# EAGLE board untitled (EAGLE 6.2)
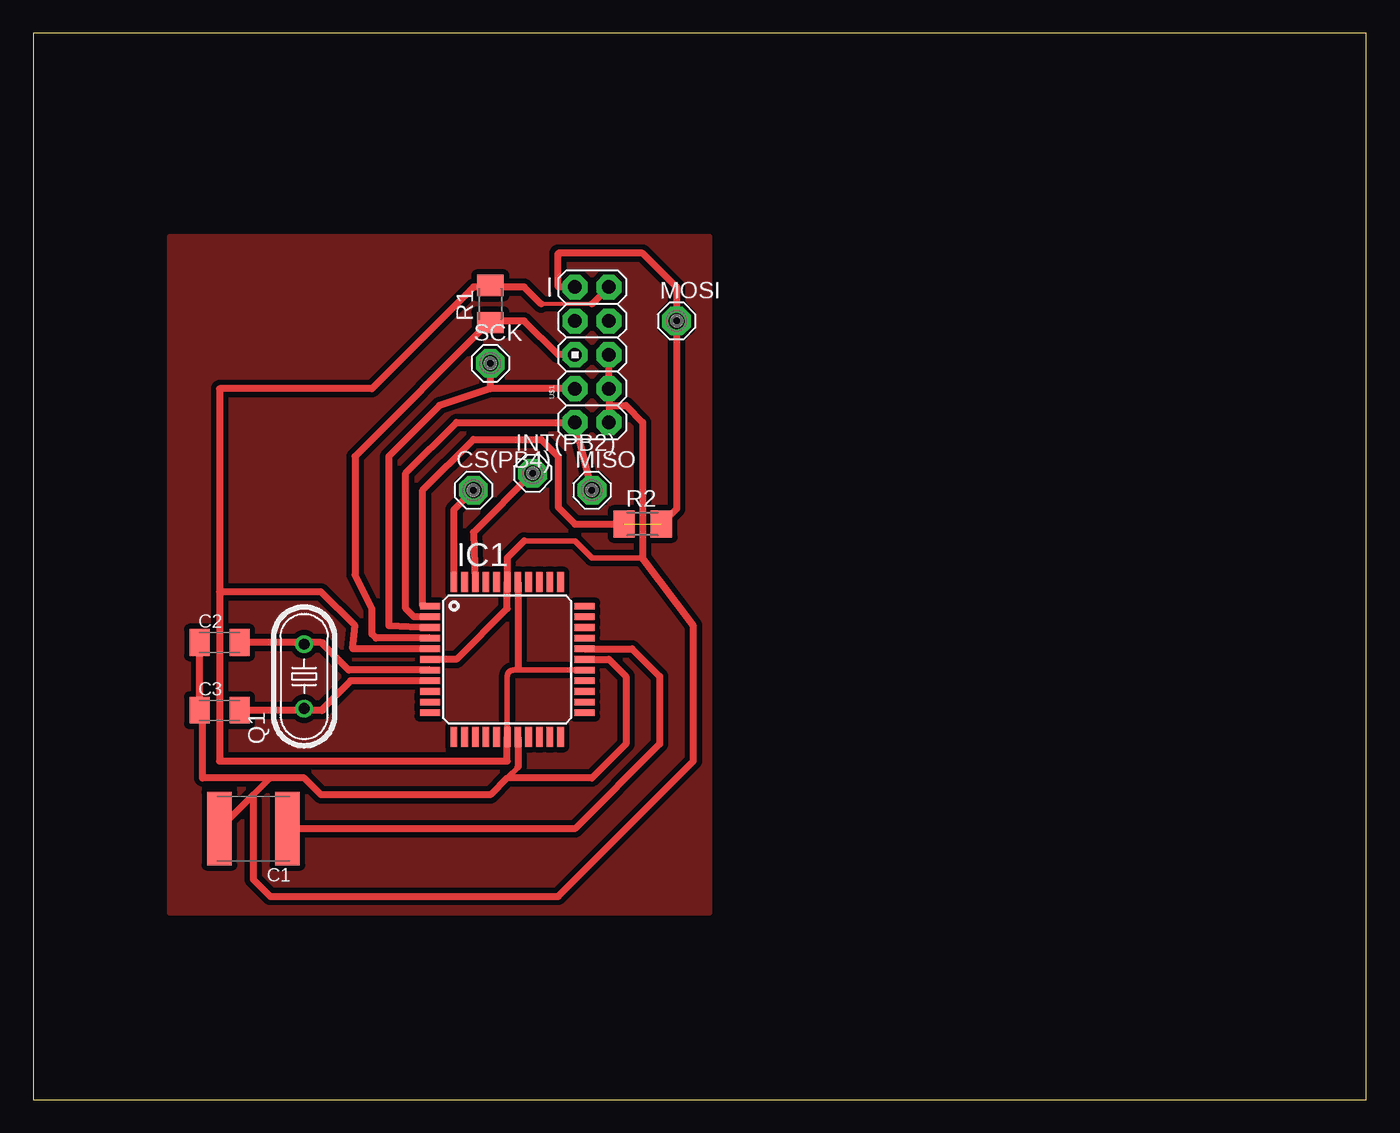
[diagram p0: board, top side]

Size 100 x 80 mm. Coordinates in mm from the lower left corner, seen from the top.
Outline: 0,0 100,0 100,80 0,80 0,0
Copper layers (1*16): Top 0.035mm / dielectric 1.5mm / Bottom 0.035mm
Design rules: minimum track width 10mil, minimum drill 24mil, track to track 8mil, track to pad 8mil, pad to pad 8mil, via to via 8mil, smd to smd 8mil, copper to edge 40mil, drill to drill 8mil, minimum pad ring 10mil, minimum via ring 8mil, stop-mask expansion 4mil, vias tented up to drill 0mil, thermal gap 10mil

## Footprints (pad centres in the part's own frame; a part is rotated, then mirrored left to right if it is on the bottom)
C2220K = smd 1.85 x 5.5: 1 -2.55,0; 2 2.55,0
C1206K = smd 1.5 x 2: 1 -1.5,0; 2 1.5,0
MCS08 = drill 1.194 pad 2.159 octagon: MP 0,0
TQFP44 = smd 1.5 x 0.5: 1 -5.8,4; 2 -5.8,3.2; 3 -5.8,2.4; 4 -5.8,1.6; 5 -5.8,0.8; 6 -5.8,0; 7 -5.8,-0.8; 8 -5.8,-1.6; 9 -5.8,-2.4; 10 -5.8,-3.2; 11 -5.8,-4; 23 5.8,-4; 24 5.8,-3.2; 25 5.8,-2.4; 26 5.8,-1.6; 27 5.8,-0.8; 28 5.8,0; 29 5.8,0.8; 30 5.8,1.6; 31 5.8,2.4; 32 5.8,3.2; 33 5.8,4 | smd 0.5 x 1.5: 12 -4,-5.8; 13 -3.2,-5.8; 14 -2.4,-5.8; 15 -1.6,-5.8; 16 -0.8,-5.8; 17 0,-5.8; 18 0.8,-5.8; 19 1.6,-5.8; 20 2.4,-5.8; 21 3.2,-5.8; 22 4,-5.8; 34 4,5.8; 35 3.2,5.8; 36 2.4,5.8; 37 1.6,5.8; 38 0.8,5.8; 39 0,5.8; 40 -0.8,5.8; 41 -1.6,5.8; 42 -2.4,5.8; 43 -3.2,5.8; 44 -4,5.8
HC49U-V = drill 0.813: 1 -2.413,0; 2 2.413,0
M1206 = smd 1.6 x 2: 1 -1.4,0; 2 1.4,0
AVR_ICSP = drill 1.016 pad 1.88 octagon: 1 -1.27,5.08; 2 1.27,5.08; 3 -1.27,2.54; 4 1.27,2.54; 5 -1.27,0; 6 1.27,0; 7 -1.27,-2.54; 8 1.27,-2.54; 9 -1.27,-5.08; 10 1.27,-5.08

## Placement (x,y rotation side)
C1  [C2220K]  16.51,20.32 180 top
C2  [C1206K]  13.97,34.29 0 top
C3  [C1206K]  13.97,29.21 0 top
CS(PB4)  MCS08  [MCS08]  33.02,45.72 0 top
IC1  MEGA32-A  [TQFP44]  35.56,33.02 0 top
INT(PB2)  MCS08  [MCS08]  37.47,46.99 0 top
MISO  MCS08  [MCS08]  41.91,45.72 0 top
MOSI  MCS08  [MCS08]  48.26,58.42 0 top
Q1  [HC49U-V]  20.32,31.75 90 top
R1  10k  [M1206]  34.29,59.69 90 top
R2  0R  [M1206]  45.72,43.18 0 top
SCK  MCS08  [MCS08]  34.29,55.24 0 top
U$1  AVR_SPI_PROG  [AVR_ICSP]  41.91,55.88 0 top

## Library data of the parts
C1-C3 R1 R2 = rcl
CS(PB4) INT(PB2) MISO MOSI SCK = solpad
IC1 = avr-7
Q1 = crystal; OC_FARNELL: 1666969; OC_NEWARK: unknown
U$1 = SparkFun

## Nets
3.3V: IC1.5 IC1.17 IC1.27 IC1.38 R1.2 U$1.2
GND: C1.2 C2.1 C3.1 IC1.6 IC1.18 IC1.28 IC1.39 U$1.6 U$1.8 U$1.10
N$1: IC1.42 INT(PB2).MP
N$2: CS(PB4).MP IC1.44
N$3: C1.1 IC1.29
N$4: C2.2 IC1.7 Q1.2
N$5: C3.2 IC1.8 Q1.1
N$6: IC1.4 R1.1 U$1.5
N$8: IC1.1 MOSI.MP R2.1 R2.2 U$1.1
N$10: IC1.3 SCK.MP U$1.7
N$11: IC1.2
S$1: U$1.9

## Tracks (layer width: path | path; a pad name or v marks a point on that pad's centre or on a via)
3.3V
  Top 0.254: 34.29,60.96 R1.2
  Top 0.305: 41.91,59.69 38.1,59.69
  Top 0.406: IC1.27 36.2,32.22 | 36.2,32.22 36.03,32.22 arc90 35.56,31.75 IC1.17 | 36.36,32.38 36.2,32.22 | 34.42,60.96 R1.2
  Top 0.508: IC1.17 35.56,25.4 13.97,25.4 13.97,38.1 | 13.97,38.1 13.97,53.34 25.4,53.34 33.02,60.96 34.29,60.96 | 41.91,59.69 U$1.2 | IC1.38 36.36,32.38 | 38.1,59.69 36.83,60.96 34.42,60.96 | IC1.5 23.96,33.82 24.13,35.56 21.59,38.1 13.97,38.1
GND
  Top 0.406: 36.36,24.93 35.56,24.13 | 17.78,24.13 16.51,22.86 16.5,22.86 | 12.7,28.98 C3.1 | 45.72,40.64 41.91,40.64 40.64,41.91 36.83,41.91
  Top 0.508: 43.18,52.07 U$1.8 U$1.6 | 43.18,52.07 U$1.10 | IC1.6 31.75,33.02 35.56,36.83 IC1.39 35.56,40.64 36.83,41.91 | IC1.18 36.36,24.93 | 16.51,22.86 16.51,16.51 17.78,15.24 39.37,15.24 49.53,25.4 49.53,35.56 45.72,40.64 45.72,50.8 44.45,52.07 43.18,52.07 | IC1.28 43.18,33.02 44.45,31.75 44.45,26.67 41.91,24.13 35.56,24.13 34.29,22.86 21.59,22.86 20.32,24.13 17.78,24.13 12.7,24.13 12.7,28.98 | C3.1 C2.1 | 16.5,22.86 C1.2
N$1
  Top 0.508: IC1.42 33.02,42.55 INT(PB2).MP
N$2
  Top 0.508: IC1.44 31.56,44.26 CS(PB4).MP
N$3
  Top 0.508: IC1.29 44.92,33.82 46.99,31.75 46.99,26.67 40.64,20.32 C1.1
N$4
  Top 0.254: 15.24,34.29 C2.2 | 21.59,34.29 Q1.2
  Top 0.406: 21.72,34.29 Q1.2
  Top 0.508: 21.59,34.29 C2.2 | IC1.7 23.66,32.22 21.59,34.29 | 21.59,34.29 21.72,34.29
N$5
  Top 0.254: 15.24,29.21 C3.2 | 21.59,29.21 Q1.1
  Top 0.406: 21.72,29.21 Q1.1
  Top 0.508: 21.59,29.21 C3.2 | IC1.8 23.8,31.42 21.59,29.21 | 21.59,29.21 21.72,29.21
N$6
  Top 0.254: 34.29,58.42 R1.1
  Top 0.508: 34.29,58.42 36.83,58.42 39.37,55.88 U$1.5 | IC1.4 25.7,34.62 25.4,34.92 25.4,36.83 24.13,39.37 24.13,48.26 34.16,58.29 R1.1
N$8  (1 unrouted)
  Top 0.406: IC1.1 29.21,37.02
  Top 0.508: U$1.1 39.37,60.96 39.37,63.5 45.72,63.5 48.26,60.96 MOSI.MP 48.26,44.32 R2.2 | 29.21,37.02 29.21,45.72 33.02,49.53 38.1,49.53 39.37,48.26 39.37,44.45 40.64,43.18 R2.1
N$10
  Top 0.508: U$1.7 34.29,53.34 | 34.29,53.34 30.48,52.07 26.67,48.26 26.67,35.56 IC1.3 | 34.29,53.34 SCK.MP
N$11
  Top 0.508: IC1.2 28.55,36.22 27.94,36.83 27.94,46.99 31.75,50.8 40.64,50.8
S$1
  Top 0.508: 41.91,45.72 U$1.9
S$2
  pour Top (isolate 0.406): 11.43,13.97 50.8,13.97 50.8,64.77 11.43,64.77 10.16,64.77 10.16,13.97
